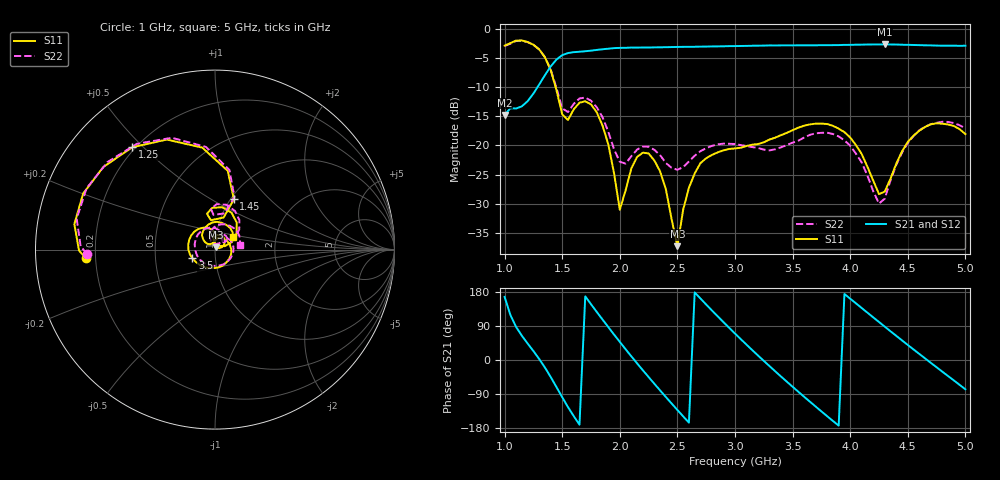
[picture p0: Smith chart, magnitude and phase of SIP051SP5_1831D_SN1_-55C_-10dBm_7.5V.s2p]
# GHz  S  dB  R  50
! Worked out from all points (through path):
!   81 points, 1 GHz to 5 GHz, reference 50 ohm
!   highest |S21| = -2.64 dB at 4.3 GHz (marker M1); lowest = -14.7 dB at 1 GHz (marker M2)
!   lowest |S11| = -37.3 dB at 2.5 GHz (marker M3), VSWR 1.03, Z = 50.4 + j1.3 ohm
!   |S11| at or under -10 dB: 1.443 GHz to end of sweep
!   |S22| runs from -30.0 to -2.0 dB; largest |S21 - S12| = 0.0022
!   S11 on the Smith chart (normalised r, x): 1 GHz: 0.16, -0.03; 1.25 GHz: 0.19, +0.46; 1.45 GHz: 1.04, +0.64; 3.5 GHz: 0.77, -0.08; 5 GHz: 1.21, +0.18
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1  -2.85 -176.2  -14.74 166.5  -14.74 166.3  -2.93 -178.0
1.15  -1.96 157.0  -13.27 63.9  -13.28 63.8  -2.02 154.5
1.25  -2.69 129.0  -11.08 23.6  -11.10 23.6  -2.70 126.5
1.45  -10.47 69.4  -5.24 -71.4  -5.23 -71.4  -10.11 69.7
1.55  -15.62 97.7  -4.12 -124.1  -4.12 -124.0  -14.25 92.4
1.7  -12.41 80.5  -3.81 167.9  -3.81 168.0  -11.77 75.4
1.9  -19.80 23.8  -3.37 86.9  -3.35 87.0  -17.63 32.0
2  -31.04 51.3  -3.23 47.8  -3.22 47.8  -22.80 43.8
2.1  -23.95 97.9  -3.18 9.7  -3.19 9.8  -21.85 65.8
2.35  -24.45 30.0  -3.13 -80.3  -3.13 -80.3  -21.67 38.9
2.5  -37.30 71.0  -3.07 -131.9  -3.07 -131.9  -24.17 46.5
2.7  -23.03 70.5  -3.02 162.3  -3.02 162.3  -20.98 46.2
2.85  -21.18 18.9  -2.98 115.2  -2.98 115.1  -19.82 23.4
3  -20.51 -32.1  -2.92 69.8  -2.91 69.7  -19.75 -5.8
3.25  -19.46 -105.2  -2.84 -2.3  -2.83 -2.3  -20.71 -74.5
3.5  -17.38 -159.1  -2.80 -70.6  -2.80 -70.6  -19.51 -162.5
3.7  -16.25 159.5  -2.79 -122.8  -2.79 -122.8  -17.91 137.6
4  -18.62 101.7  -2.71 161.8  -2.72 161.8  -20.03 69.5
4.3  -27.92 131.2  -2.64 88.0  -2.65 88.0  -29.13 104.7
4.35  -25.70 142.6  -2.65 75.8  -2.66 75.9  -26.00 115.0
4.65  -16.81 104.6  -2.79 4.3  -2.80 4.2  -16.78 76.6
5  -18.05 35.2  -2.86 -77.3  -2.87 -77.3  -17.03 11.2
